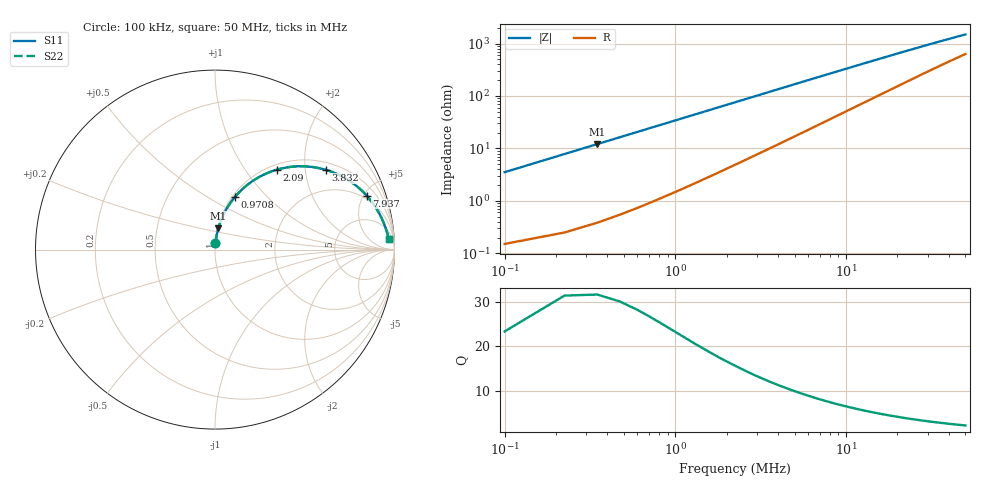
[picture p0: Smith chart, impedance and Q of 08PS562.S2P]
! Coilcraft 0805PS-562 Power Chip Inductor
! 5 February 2003
# MHZ S MA R 50
!Freq  MagS11  AngS11  MagS21  AngS21  MagS12  AngS12  MagS22  AngS22
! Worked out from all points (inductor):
!   403 points, 100 kHz to 50 MHz, reference 50 ohm
!   read as one part in series: L = 5.51 uH near 348.8 kHz
!   highest Q = 26.5 at 348.8 kHz (marker M1), where L = 5.53 uH
!   S11 on the Smith chart (normalised r, x): 100 kHz: 1.00, +0.07; 970.8 kHz: 1.03, +0.67; 2.09 MHz: 1.09, +1.42; 3.832 MHz: 1.22, +2.58; 7.937 MHz: 1.70, +5.24; 50 MHz: 14, +27
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0.1  0.03514 85.5  0.9979 -2.0  0.9979 -2.0  0.03514 85.5
0.2244  0.07791 83.7  0.9945 -4.5  0.9945 -4.5  0.07791 83.7
0.3488  0.1199 81.3  0.989 -6.9  0.989 -6.9  0.1199 81.3
0.4732  0.1609 78.8  0.9816 -9.3  0.9816 -9.3  0.1609 78.8
0.5976  0.2008 76.4  0.9726 -11.6  0.9726 -11.6  0.2008 76.4
0.722  0.2394 74.0  0.9619 -13.8  0.9619 -13.8  0.2394 74.0
0.9708  0.3124 69.4  0.9368 -18.2  0.9368 -18.2  0.3124 69.4
1.2196  0.3793 65.0  0.9076 -22.3  0.9076 -22.3  0.3793 65.0
1.4684  0.4397 61.0  0.8758 -26.0  0.8758 -26.0  0.4397 61.0
2.0904  0.5636 52.2  0.792 -34.2  0.792 -34.2  0.5636 52.2
2.9612  0.6832 42.8  0.681 -42.9  0.681 -42.9  0.6832 42.8
3.832  0.76 35.8  0.5876 -49.2  0.5876 -49.2  0.76 35.8
4.7028  0.8105 30.6  0.5122 -53.8  0.5122 -53.8  0.8105 30.6
5.5736  0.8448 26.7  0.4518 -57.1  0.4518 -57.1  0.8448 26.7
7.9372  0.8967 19.6  0.3391 -62.7  0.3391 -62.7  0.8967 19.6
8.4348  0.9033 18.6  0.3219 -63.5  0.3219 -63.5  0.9033 18.6
12.1668  0.933 13.2  0.2327 -66.8  0.2327 -66.8  0.933 13.2
16.7696  0.9486 9.8  0.1736 -68.0  0.1736 -68.0  0.9486 9.8
25.1044  0.9604 6.6  0.1199 -67.4  0.1199 -67.4  0.9604 6.6
33.4392  0.9657 5.0  0.09244 -65.7  0.09244 -65.7  0.9657 5.0
41.774  0.9687 4.0  0.07592 -63.7  0.07592 -63.7  0.9687 4.0
50  0.9707 3.4  0.06504 -61.6  0.06504 -61.6  0.9707 3.4
